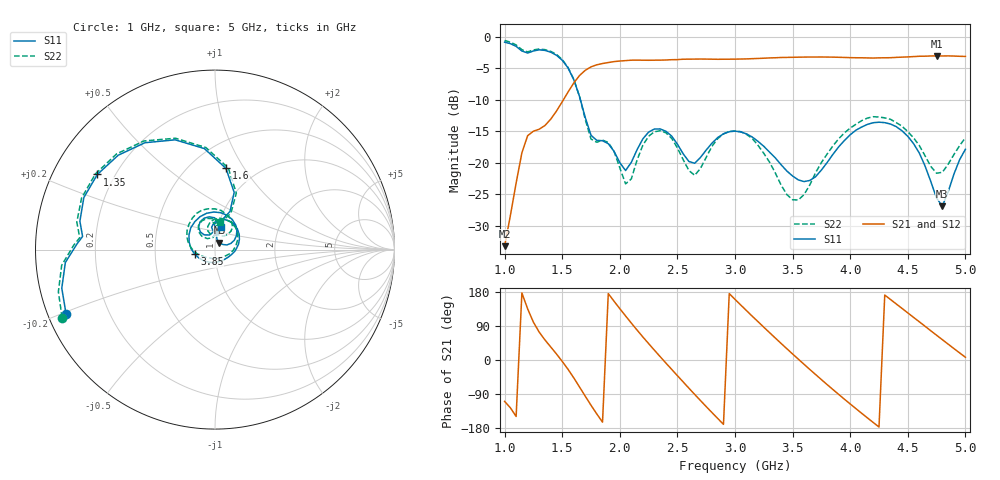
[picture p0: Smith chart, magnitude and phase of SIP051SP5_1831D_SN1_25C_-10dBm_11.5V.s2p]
# GHz  S  dB  R  50
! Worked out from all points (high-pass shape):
!   81 points, 1 GHz to 5 GHz, reference 50 ohm
!   highest |S21| = -3.05 dB at 4.75 GHz (marker M1); lowest = -33.2 dB at 1 GHz (marker M2)
!   |S21| within 3 dB of the highest: 1.657 GHz to end of sweep
!   lowest |S11| = -26.9 dB at 4.8 GHz (marker M3), VSWR 1.09, Z = 52.4 + j3.97 ohm
!   |S11| at or under -10 dB: 1.658 GHz to end of sweep
!   |S22| runs from -25.9 to -0.6 dB; largest |S21 - S12| = 0.003
!   S11 on the Smith chart (normalised r, x): 1 GHz: 0.05, -0.21; 1.35 GHz: 0.14, +0.29; 1.6 GHz: 0.73, +0.83; 3.85 GHz: 0.79, -0.04; 5 GHz: 1.03, +0.26
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1  -0.88 -156.7  -33.23 -109.2  -33.40 -108.7  -0.61 -156.0
1.15  -2.27 177.6  -18.43 176.9  -18.41 176.8  -2.07 178.3
1.35  -2.18 147.4  -14.09 53.0  -14.08 53.1  -2.06 147.7
1.5  -3.73 109.9  -10.33 -3.6  -10.32 -3.4  -3.63 109.5
1.6  -6.81 82.3  -7.37 -47.0  -7.36 -47.0  -6.73 80.7
1.7  -12.81 68.5  -5.34 -95.5  -5.33 -95.6  -13.13 66.4
1.9  -16.98 91.3  -4.11 175.2  -4.10 175.3  -16.78 89.8
2.1  -19.93 125.8  -3.73 97.5  -3.73 97.4  -22.56 124.9
2.35  -14.64 100.1  -3.73 9.0  -3.73 9.0  -14.93 104.0
2.65  -20.08 90.5  -3.56 -90.8  -3.56 -90.6  -22.00 93.5
2.85  -16.00 88.1  -3.59 -154.3  -3.59 -154.2  -16.17 100.0
3  -14.98 61.8  -3.57 160.0  -3.56 160.1  -14.95 70.2
3.3  -18.32 4.2  -3.38 72.2  -3.37 72.2  -19.90 -2.7
3.5  -22.10 -40.2  -3.28 15.9  -3.28 15.9  -25.87 -77.6
3.7  -22.21 -114.1  -3.24 -38.5  -3.23 -38.4  -21.56 -154.7
3.85  -18.66 -167.9  -3.25 -77.9  -3.25 -77.9  -17.33 174.3
4.1  -14.33 125.9  -3.36 -140.7  -3.36 -140.7  -13.32 125.9
4.35  -13.86 70.6  -3.34 159.6  -3.33 159.6  -13.12 81.4
4.55  -16.97 32.8  -3.17 112.5  -3.17 112.6  -16.04 52.1
4.75  -25.61 32.6  -3.05 65.3  -3.06 65.4  -21.66 64.6
4.8  -26.88 56.5  -3.07 53.6  -3.06 53.6  -21.51 77.1
5  -17.87 75.6  -3.14 7.3  -3.15 7.4  -16.03 78.9
